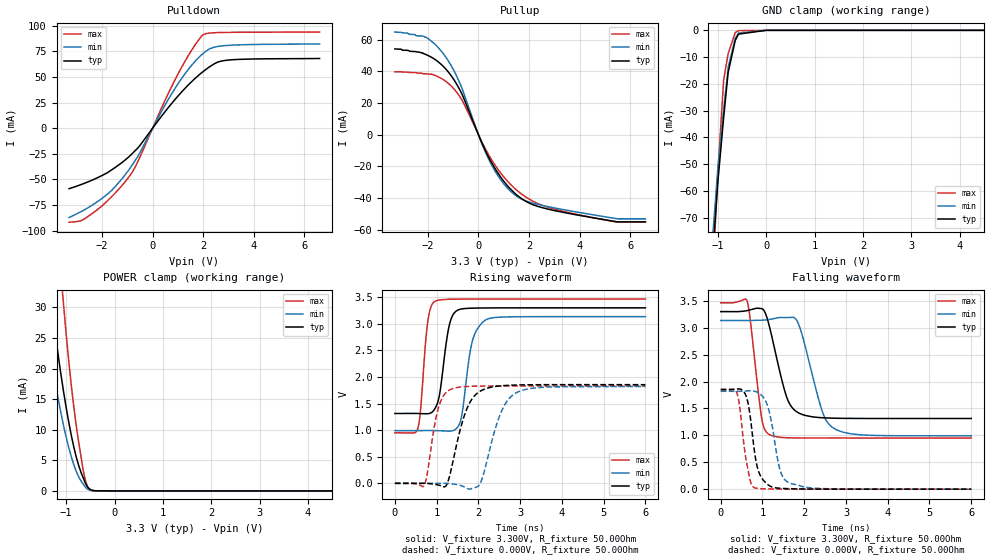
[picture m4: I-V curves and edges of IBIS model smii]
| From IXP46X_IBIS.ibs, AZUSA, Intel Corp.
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|* NOTE : The SMII Model uses a special compensation scheme, thus the
|* NOTE : Min/Typ/Max curves are not ordered in the conventional way.
|* NOTE : For Pullups, MIN has the highest drive current and
|* NOTE : MAX has the lowest drive current.
|* NOTE : For pulldowns, MAX has the highest drive current and
|* NOTE : TYP has the lowest drive current.
|* NOTE : It is Recommended that Signal Integrity simulations
|* NOTE : be carried out to cover all the corner conditions.
|* NOTE :
[Model]   smii
Model_type   I/O
Vinl = 800.000mV
Vinh = 2.000V
Vmeas = 1.500V
Cref = 0.000F
|   typ   min   max
C_comp   3.000pF   2.700pF   3.300pF
[Voltage Range]   3.300V   3.135V   3.465V
[Temperature Range]   25.0   110.0   -40.0
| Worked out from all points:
|   slope of the pulldown table from 0 to 0.495 V, typ, clamps not added: 30.6 ohm
|   slope of the pullup table from 0 to 0.495 V, typ, clamps not added: 29.3 ohm
|   POWER clamp passes 1 mA (typ) near -0.59 V on its own axis
|   falling waveform, V_fixture 3.300V, R_fixture 50.00Ohm: 20-80 % time 376ps typ, 439ps min, 221ps max; typ from 3.3 V to 1.31 V
|   rising waveform, V_fixture 3.300V, R_fixture 50.00Ohm: 20-80 % time 206ps typ, 237ps min, 154ps max; typ from 1.31 V to 3.3 V
|   rising waveform, V_fixture 0.000V, R_fixture 50.00Ohm: 20-80 % time 392ps typ, 430ps min, 249ps max; typ from 0 V to 1.85 V
|   falling waveform, V_fixture 0.000V, R_fixture 50.00Ohm: 20-80 % time 209ps typ, 261ps min, 189ps max; typ from 1.85 V to 0 V
[Pulldown]
|   Voltage   I(typ)   I(min)   I(max)
-3.3V     -59.02mA   -87.14mA   -91.69mA
-2.835V   -55.06mA   -81.52mA   -90.21mA
-2.305V   -49.75mA   -73.78mA   -81.77mA
-1.605V   -40.45mA   -60.36mA   -66.41mA
-920mV    -27.52mA   -40.03mA   -46.98mA
-605mV    -19.87mA   -28.35mA   -33.74mA
890mV     28.14mA    39mA       47.43mA
1.5V      44.39mA    60.15mA    74.39mA
1.99V     55.15mA    72.74mA    90.98mA
2.29V     60.53mA    77.82mA    92.88mA
2.875V    66.15mA    80.61mA    93.44mA
6.595V    67.99mA    82.18mA    93.77mA
[GND Clamp]
|   Voltage   I(typ)   I(min)   I(max)
-3.3V     -1.837A    -1.782A    -2.189A
-1.1V     -82.07mA   -75.29mA   -89.82mA
-1.005V   -57.88mA   -52.75mA   -54.99mA
-995mV    -55.65mA   -50.66mA   -51.64mA
-880mV    -32.52mA   -29.52mA   -18.54mA
-785mV    -15.53mA   -13.67mA   -8.623mA
-640mV    -3.748mA   -2.925mA   -837uA
-575mV    -1.514mA   -1.11mA    -135.3uA
0V        -56.84nA   -17.58nA   -565.5pA
6.595V    0A         0A         0A
[Pullup]
|   Voltage   I(typ)   I(min)   I(max)
-3.3V     54.13mA    64.75mA    39.72mA
-2.205V   51.59mA    62.33mA    38.62mA
-1.39V    43.14mA    51.19mA    34.78mA
-670mV    26.22mA    30.05mA    22.38mA
95mV      -3.65mA    -4.031mA   -3.256mA
470mV     -16.17mA   -17.56mA   -14.49mA
980mV     -28.98mA   -30.62mA   -26.25mA
1.465V    -37.38mA   -38.32mA   -34.39mA
2.105V    -43.9mA    -43mA      -41.6mA
3.05V     -48.08mA   -46.42mA   -47.21mA
5.5V      -55.05mA   -53.13mA   -55.25mA
6.595V    -55.05mA   -53.13mA   -55.25mA
[POWER Clamp]
|   Voltage   I(typ)   I(min)   I(max)
-3.3V     221.1mA    178.3mA    361mA
-1.505V   44.7mA     32.22mA    80.58mA
-1.325V   32.02mA    22.46mA    58.62mA
-1.085V   17.79mA    11.8mA     33.27mA
-1.065V   16.76mA    11.05mA    31.4mA
-930mV    10.52mA    6.585mA    19.92mA
-855mV    7.631mA    4.595mA    14.57mA
-785mV    5.35mA     3.076mA    10.29mA
-640mV    2mA        1.037mA    3.043mA
-540mV    479.4uA    207uA      465.4uA
-390mV    28.44uA    11.22uA    5.344uA
6.595V    0A         0A         0A
[Ramp]
R_load = 50.00Ohm
|   typ   min   max
dV/dt_r   1.113V/391.486ps   1.092V/428.625ps   1.099V/248.259ps
dV/dt_f   1.192V/375.896ps   1.286V/437.858ps   1.509V/220.635ps
[Falling Waveform]
V_fixture = 3.300V
V_fixture_min = 3.135V
V_fixture_max = 3.465V
R_fixture = 50.00Ohm
|   Time   V(typ)   V(min)   V(max)
0s        3.3V       3.135V     3.465V
630ps     3.318V     3.135V     3.502V
710ps     3.333V     3.135V     3.129V
980ps     3.356V     3.141V     1.324V
1.17ns    3.012V     3.155V     1.012V
1.58ns    1.711V     3.189V     956.2mV
1.91ns    1.401V     2.969V     951.3mV
2.43ns    1.328V     1.452V     950.8mV
2.73ns    1.319V     1.121V     951.9mV
6ns       1.313V     991.4mV    949.8mV
[Rising Waveform]
V_fixture = 3.300V
V_fixture_min = 3.135V
V_fixture_max = 3.465V
R_fixture = 50.00Ohm
|   Time   V(typ)   V(min)   V(max)
0s        1.313V     991.4mV    949.8mV
550ps     1.313V     991.3mV    1.032V
790ps     1.309V     992.7mV    3.047V
960ps     1.406V     991.9mV    3.423V
1.07ns    1.672V     989.2mV    3.447V
1.31ns    2.995V     981.2mV    3.462V
1.52ns    3.262V     1.075V     3.464V
1.85ns    3.294V     2.656V     3.465V
2.15ns    3.298V     3.062V     3.465V
6ns       3.3V       3.135V     3.465V
[Rising Waveform]
V_fixture = 0.000V
V_fixture_min = 0.000V
V_fixture_max = 0.000V
R_fixture = 50.00Ohm
|   Time   V(typ)   V(min)   V(max)
0s        1.054uV    261nV      -6.12nV
700ps     33.05uV    -157.8uV   -46.01mV
1.04ns    -31.75mV   952.8uV    1.412V
1.22ns    -51.85mV   636.7uV    1.702V
1.36ns    299mV      -8.845mV   1.774V
1.71ns    1.374V     -87.21mV   1.82V
2.13ns    1.766V     192.3mV    1.829V
2.51ns    1.831V     1.273V     1.831V
2.9ns     1.849V     1.7V       1.831V
6ns       1.855V     1.819V     1.832V
[Falling Waveform]
V_fixture = 0.000V
V_fixture_min = 0.000V
V_fixture_max = 0.000V
R_fixture = 50.00Ohm
|   Time   V(typ)   V(min)   V(max)
0s        1.855V     1.819V     1.832V
390ps     1.86V      1.819V     1.782V
630ps     1.677V     1.826V     453mV
720ps     1.268V     1.829V     120.1mV
810ps     693.3mV    1.82V      26.06mV
910ps     323.5mV    1.787V     11.68mV
1.11ns    97.68mV    1.575V     5.39mV
1.41ns    17.49mV    385.6mV    1.349mV
1.66ns    8.126mV    111mV      308.7uV
6ns       1.054uV    261nV      -6.12nV
